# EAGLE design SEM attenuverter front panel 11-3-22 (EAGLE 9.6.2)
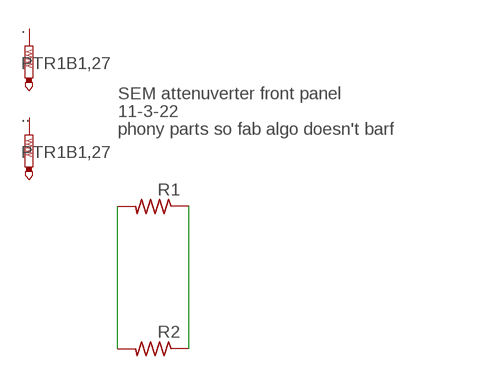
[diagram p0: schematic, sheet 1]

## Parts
.  PTR1B1,27  [B1,27]
..  PTR1B1,27  [B1,27]
R1  R-US_M0805  [M0805]
R2  R-US_M0805  [M0805]

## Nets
N$1: R1.2 R2.2
N$2: R1.1 R2.1
Unconnected: ...TP ..TP

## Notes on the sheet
- SEM attenuverter front panel
- 11-3-22
- phony parts so fab algo doesn't barf

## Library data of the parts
. .. = testpad:PTR1: TEST PIN
R1 R2 = adafruit:R-US_: RESISTOR, American symbol

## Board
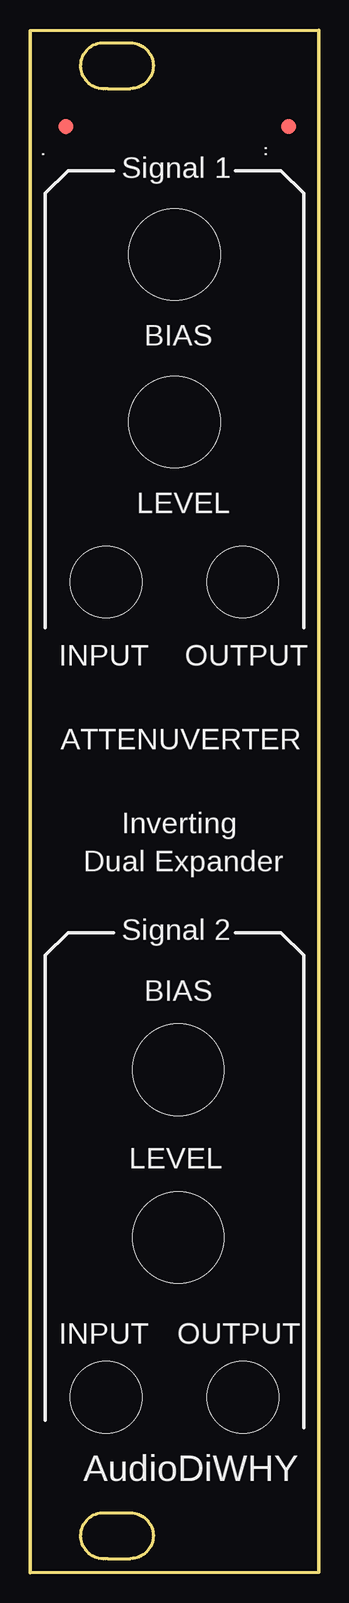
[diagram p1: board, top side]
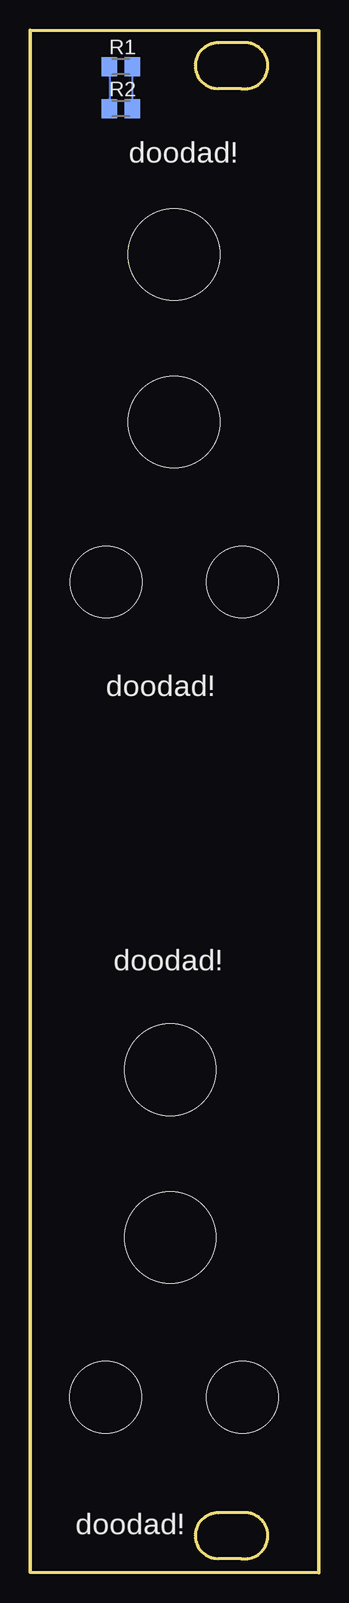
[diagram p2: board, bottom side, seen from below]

Size 24.09 x 128.56 mm. Coordinates in mm from the lower left corner, seen from the top.
Outline: 0,0 24.09,0.06 24.09,128.56 0,128.5 0,0
Copper layers (1*16): Top 0.035mm / dielectric 1.5mm / Bottom 0.035mm
Design rules "default": minimum track width 6mil, minimum drill 0.35mm, track to track 6mil, track to pad 6mil, pad to pad 6mil, via to via 6mil, smd to smd 6mil, copper to edge 40mil, drill to drill 6mil, minimum pad ring 10mil, minimum via ring 8mil, stop-mask expansion 4mil, vias tented up to drill 0mil, thermal gap 10mil
Holes 5.97 mm at 6.35,14.61 6.35,82.55 17.78,14.61 17.75,82.55
Holes 7.62 mm at 12.38,27.94 12.38,41.91 12.06,95.89 12.06,109.86
Milling: 8 lines

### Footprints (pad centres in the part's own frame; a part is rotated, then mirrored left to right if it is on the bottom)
B1,27 = smd 1.27 x 1.27: TP 0,0
M0805 = smd 1.3 x 1.6: 1 -0.95,0; 2 0.95,0

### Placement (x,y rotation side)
.  3,120.5 0 top
..  21.58,120.5 0 top
R1  16.5,125.5 0 bottom
R2  16.5,122 0 bottom

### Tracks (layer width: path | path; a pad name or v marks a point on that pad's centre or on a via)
N$1
  Bottom 0.152: R1.2 R2.2
N$2
  Bottom 0.152: R1.1 R2.1

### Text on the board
tNames: Signal 1 | BIAS | LEVEL | INPUT | OUTPUT | ATTENUVERTER | Inverting | Dual Expander | Signal 2 | BIAS | LEVEL | INPUT | OUTPUT | AudioDiWHY
bNames: doodad! | doodad! | doodad! | doodad!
